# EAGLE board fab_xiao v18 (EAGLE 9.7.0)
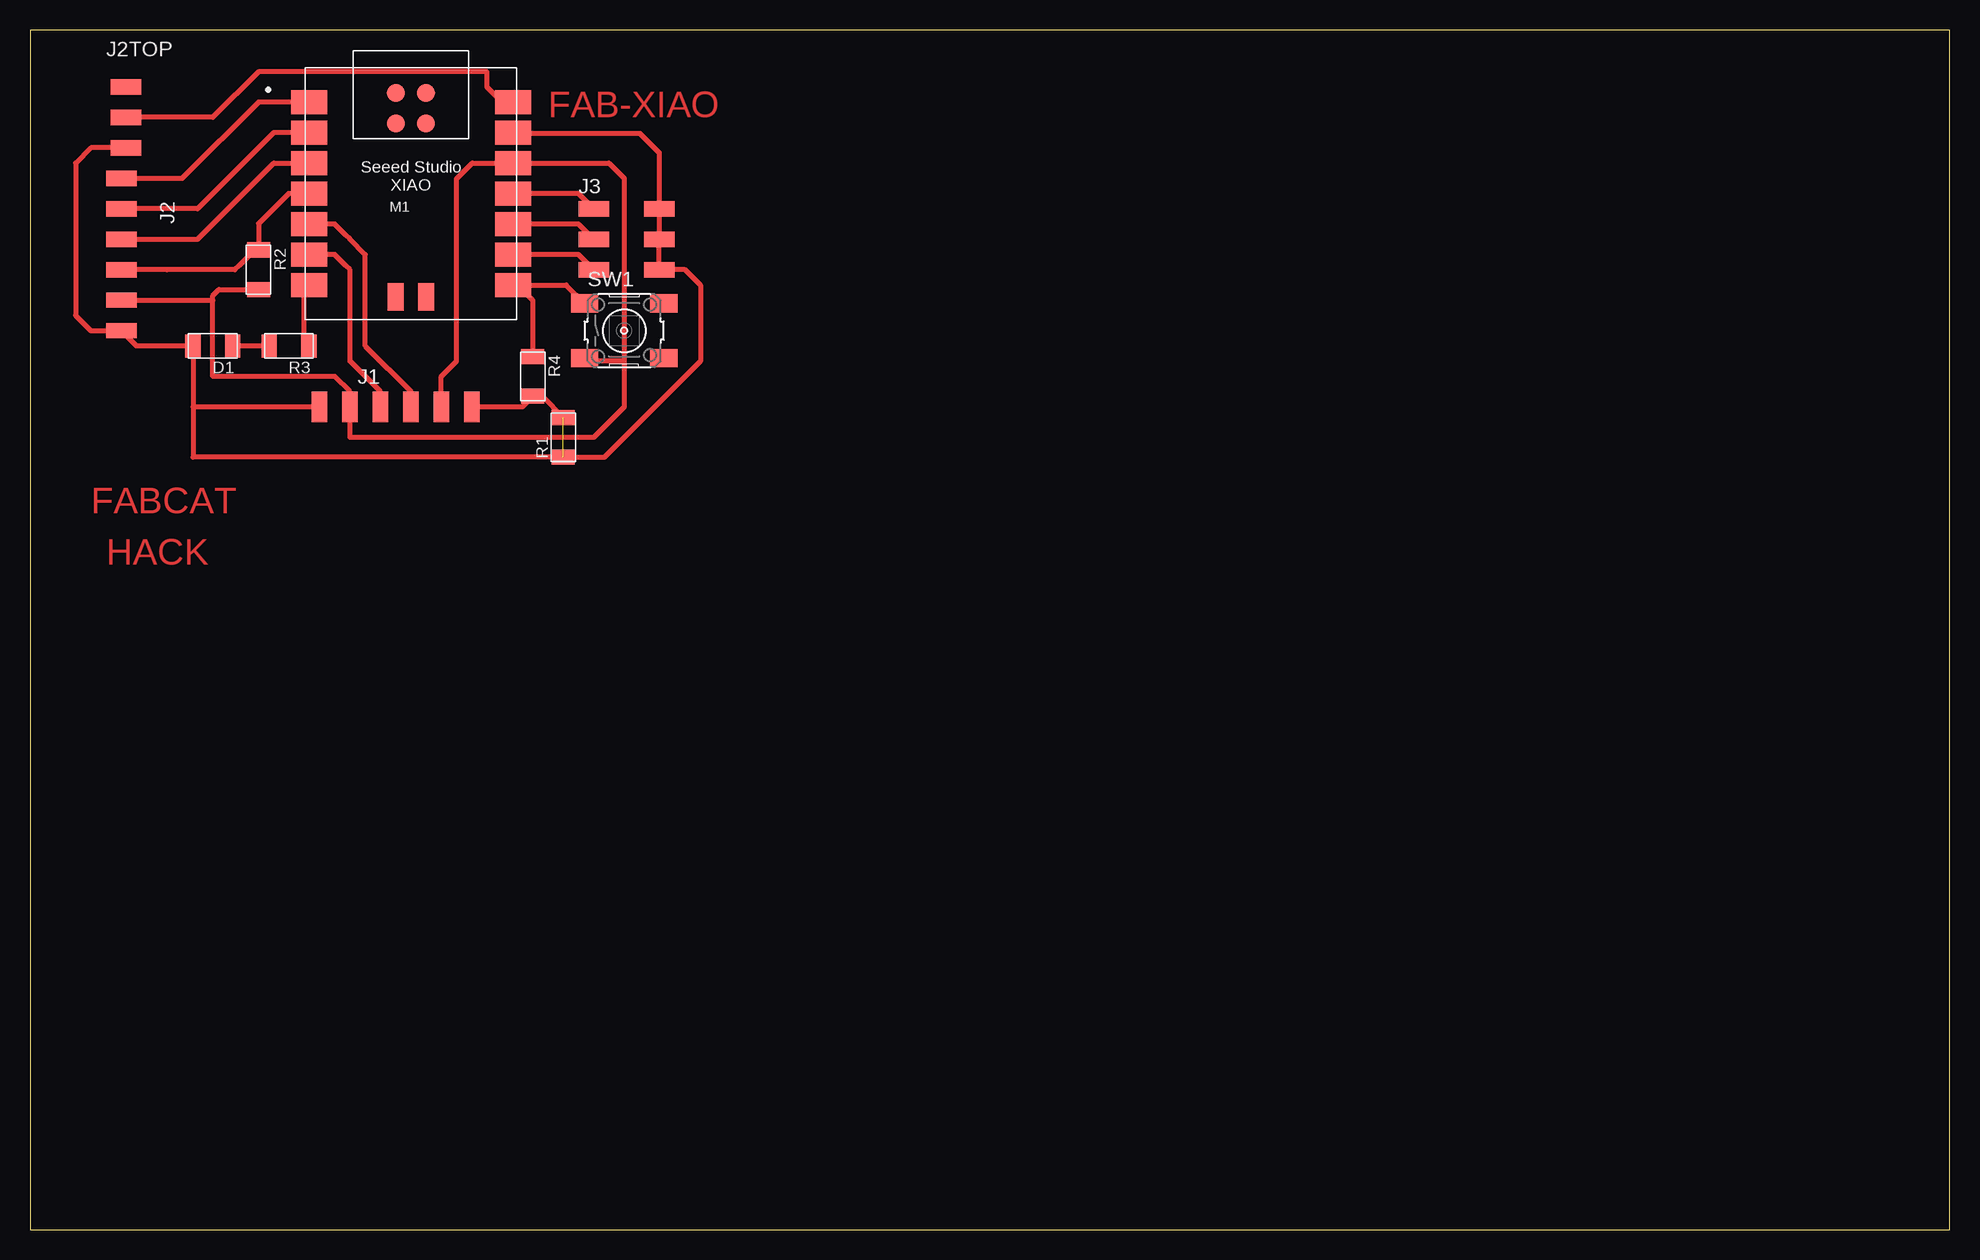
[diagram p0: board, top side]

Size 160 x 100 mm. Coordinates in mm from the lower left corner, seen from the top.
Outline: 0,0 160,0 160,100 0,100 0,0
Copper layers (1*16): Top 0.035mm / dielectric 1.5mm / Bottom 0.035mm
Design rules "default *": minimum track width 16mil, minimum drill 0.35mm, track to track 16mil, track to pad 16mil, pad to pad 16mil, via to via 16mil, smd to smd 6mil, copper to edge 40mil, drill to drill 6mil, minimum pad ring 10mil, minimum via ring 8mil, stop-mask expansion 4mil, vias tented up to drill 0mil, thermal gap 10mil

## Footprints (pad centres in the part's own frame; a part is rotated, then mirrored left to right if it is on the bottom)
LED1206FAB = smd 1.27 x 1.905: 1 -1.651,0; 2 1.651,0
1X06SMD = smd 2.54 x 1.27: 1 0,6.35; 2 0,3.81; 3 0,1.27; 4 0,-1.27; 5 0,-3.81; 6 0,-6.35
SPDTSWITCH = smd 2.54 x 1.27: 1 0.38,2.54; 2 0.38,0; 3 0.38,-2.54
2X03SMD = smd 2.54 x 1.27: 1 -2.54,2.54; 2 2.92,2.54; 3 -2.54,0; 4 2.92,0; 5 -2.54,-2.54; 6 2.92,-2.54
XIAO-SAMD21/RP2040-MODULE14P-2.54-21X17.8MM = smd 3 x 2: 1 -8.5,7.62; 2 -8.5,5.08; 3 -8.5,2.54; 4 -8.5,0; 5 -8.5,-2.54; 6 -8.5,-5.08; 7 -8.5,-7.62; 8 8.5,-7.62; 9 8.5,-5.08; 10 8.5,-2.54; 11 8.5,0; 12 8.5,2.54; 13 8.5,5.08; 14 8.5,7.62 | smd 1.5 x 1.5: 15 -1.27,8.39; 16 1.27,8.39; 17 -1.27,5.85; 18 1.27,5.85 | smd 1.3 x 2.3: 19 -1.27,-8.6; 20 1.27,-8.6
R1206FAB = smd 1.27 x 1.905: 1 -1.651,0; 2 1.651,0
6MM_SWITCH = smd 2.286 x 1.524: 1 -3.302,2.286; 2 3.302,2.286; 3 -3.302,-2.286; 4 3.302,-2.286

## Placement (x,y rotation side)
D1  LEDFAB1206  [LED1206FAB]  15.24,73.66 180 top
J1  CONN_06_FTDI-SMD-HEADER  [1X06SMD]  30.48,68.58 270 top
J2  CONN_06_FTDI-SMD-HEADER  [1X06SMD]  7.62,81.28 180 top
J2TOP  SPDTSWITCH  [SPDTSWITCH]  7.62,92.71 0 top
J3  [2X03SMD]  49.53,82.55 0 top
M1  XIAO-RP2040  [XIAO-SAMD21/RP2040-MODULE14P-2.54-21X17.8MM]  31.75,86.36 0 top
R1  0  [R1206FAB]  44.45,66.04 90 top
R2  4.7K  [R1206FAB]  19.05,80.01 270 top
R3  1K  [R1206FAB]  21.59,73.66 180 top
R4  470  [R1206FAB]  41.91,71.12 270 top
SW1  [6MM_SWITCH]  49.53,74.93 0 top

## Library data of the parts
D1 J1 J2 J2TOP J3 R1-R4 SW1 = fab
M1 = Seeed Studio XIAO Series

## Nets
3V3: J1.2 J1.5 J2.2 M1.12 R2.2 SW1.3
5V [New Class]: J2TOP.2 M1.14
A0: J2.6 M1.1
A1: J2.5 M1.2
A2: J2.4 M1.3
A3: J2.3 M1.4 R2.1
A6: M1.7 R3.1
A7: M1.8 R4.1 SW1.1
A8: J3.5 M1.9
A9: J3.3 M1.10
A10: J3.1 M1.11
GND: D1.2 J1.1 J1.6 J2.1 J2TOP.3 J3.2 J3.4 J3.6 M1.13 R1.1 R1.2 R4.2
N$2: J2TOP.1
N$3: D1.1 R3.2
SCL: J1.4 M1.6
SDA: J1.3 M1.5

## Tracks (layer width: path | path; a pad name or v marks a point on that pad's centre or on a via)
3V3
  Top 0.406: 49.53,72.39 46.48,72.39 SW1.3 | 49.53,72.39 49.53,87.63 48.26,88.9 M1.12 36.86,88.9 35.56,87.6 35.56,72.39 34.29,71.12 J1.2 | 49.53,72.39 49.53,68.58 46.99,66.04 26.67,66.04 J1.5 26.67,69.85 25.4,71.12 15.24,71.12 15.24,77.47 | 15.24,77.47 15.24,77.85 15.75,78.36 R2.2 | J2.2 15.24,77.47
5V
  Top 0.406: J2TOP.2 15.24,92.71 19.05,96.52 38.1,96.52 38.1,95.25 39.37,93.98 M1.14
A0
  Top 0.406: M1.1 19.05,93.98 12.7,87.63 J2.6
A1
  Top 0.406: M1.2 20.32,91.44 13.97,85.09 J2.5
A2
  Top 0.406: J2.4 13.97,82.55 20.32,88.9 M1.3
A3
  Top 0.406: M1.4 21.55,86.36 19.05,83.86 R2.1 18.73,81.66 17.43,80.36 17.08,80.01 11.43,80.01 J2.3
A6
  Top 0.406: R3.1 22.86,73.66 22.86,78.35 M1.7
A7
  Top 0.406: SW1.1 44.7,78.74 40.64,78.74 | M1.8 40.64,78.74 | 40.64,78.74 41.91,77.47 R4.1
A8
  Top 0.406: 46.65,80.35 J3.5 45.72,81.28 M1.9
A9
  Top 0.406: 46.65,82.89 J3.3 45.72,83.82 M1.10
A10
  Top 0.406: 46.65,85.43 J3.1 45.72,86.36 M1.11
GND  (1 unrouted)
  Top 0.406: J1.1 41.02,68.58 R4.2 42.67,69.47 R1.2 | J2TOP.3 5.08,90.17 3.81,88.9 3.81,76.2 5.08,74.93 J2.1 8.89,73.66 D1.2 13.59,68.58 | M1.13 40.32,91.37 50.87,91.37 52.45,89.79 J3.2 J3.4 J3.6 54.61,80.01 55.88,78.74 55.88,72.39 47.88,64.39 R1.1 13.59,64.39 13.59,68.58 | J1.6 16.51,68.58 13.59,68.58
N$3
  Top 0.406: R3.2 D1.1
SCL
  Top 0.406: J1.4 29.21,69.85 26.67,72.39 26.67,80.01 26.33,80.35 25.4,81.28 M1.6
SDA
  Top 0.406: J1.3 31.75,69.85 27.94,73.66 27.94,81.28 26.67,82.55 26.33,82.89 25.4,83.82 M1.5 22.86,83.82

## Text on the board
Top: FAB-XIAO | FABCAT | HACK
